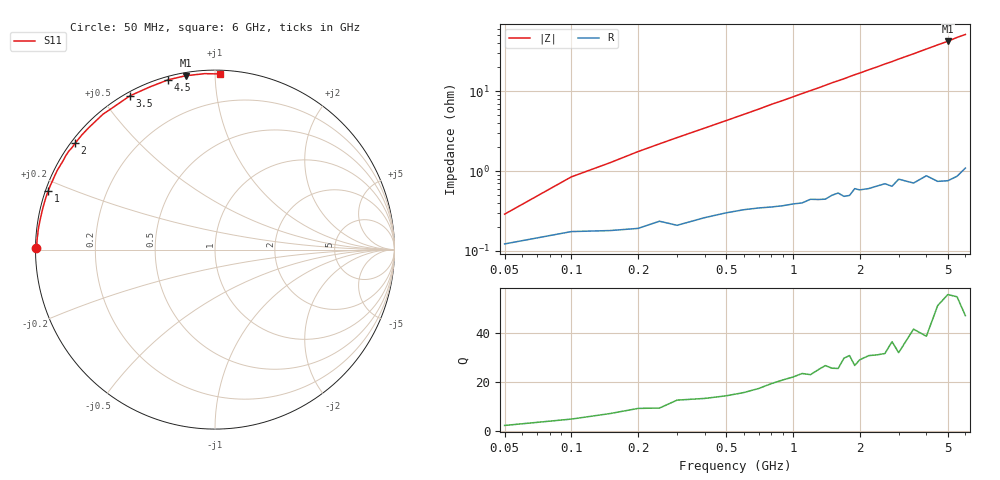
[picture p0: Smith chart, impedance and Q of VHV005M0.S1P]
! Infineon Technologies  Discrete & RF Semiconductors
! BB 814
! Si Tuning Diode in SOT23
! VR =
! S-Parameters:  July  1999
# GHz  S  MA  R  50
!  f  S11
! GHz  MAG  ANG
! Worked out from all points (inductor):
!   34 points, 50 MHz to 6 GHz, reference 50 ohm
!   read as one part to ground: L = 1.34 nH near 100 MHz
!   highest Q = 54.8 at 5 GHz (marker M1), where L = 1.34 nH
!   S11 on the Smith chart (normalised r, x): 50 MHz: 0.00, +0.01; 1 GHz: 0.01, +0.17; 2 GHz: 0.01, +0.34; 3.5 GHz: 0.01, +0.59; 4.5 GHz: 0.01, +0.76; 6 GHz: 0.02, +1.03
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0.05  0.9951 179.4
0.1  0.993 178.1
0.2  0.9924 176.0
0.25  0.9906 175.0
0.3  0.9917 174.0
0.6  0.9871 168.3
0.8  0.9861 164.4
1  0.985 160.7
1.1  0.9847 158.8
1.3  0.9833 155.2
1.4  0.9833 153.3
1.5  0.9814 151.4
1.6  0.9804 149.7
1.7  0.9823 148.0
1.8  0.982 146.1
1.9  0.9784 144.3
2  0.9793 142.7
2.2  0.9789 139.2
2.4  0.9778 136.0
2.6  0.9769 132.6
2.8  0.9791 129.6
3  0.9751 126.3
3.5  0.9792 119.0
4  0.9763 111.9
4.5  0.9813 105.4
5  0.9825 99.6
5.5  0.9819 93.3
6  0.979 88.4
